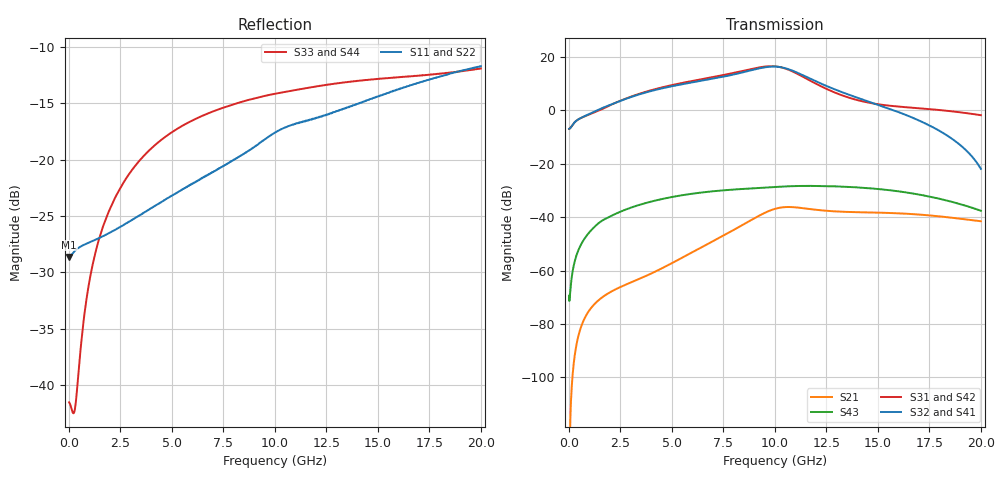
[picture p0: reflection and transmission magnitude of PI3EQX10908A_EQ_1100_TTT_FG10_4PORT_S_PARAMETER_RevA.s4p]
! NPort=4 DATA=2000 NOISE=0 GROUPDELAY=0 COMPLEX_DATAFORMAT=POLAR
! NumOfBlock=1 NumOfParam=0
! .MODEL Smodel S TSTONEFILE=PI3EQX10908A_EQ_1100_TTT_FG10_4PORT_S_PARAMETER_RevA.s4p TYPE=S
!  -- The above .MODEL line can be used for the S element in the netlist.
! The s parameter is extracted from the linear redriver, it is not bi-directional; only s(4,1)s(4,2) and s(3,1)s(3,2)
! should be the insertion loss
!Port definition:
!Port1 = input+
!Port2 = input-
!Port3 = output+
!Port4 = output-
# Hz S MA R  50
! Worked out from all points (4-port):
!   2000 points, 10 MHz to 20 GHz, reference 50 ohm
!   strongest paths, dB at 10 MHz, 5.01 GHz, 10.01 GHz, 15.01 GHz, 20 GHz:
!     S32: -6.9, 9.0, 16.4, 2.1, -21.9
!     S41: -6.9, 9.0, 16.4, 2.1, -21.9
!     S31: -6.9, 9.5, 16.5, 2.3, -1.8
!     S42: -6.9, 9.5, 16.5, 2.3, -1.8
!     S43: -69.4, -32.4, -28.7, -29.5, -37.6
!     S21: -127.3, -57.2, -36.9, -38.3, -41.5
!   lowest |S11| = -28.6 dB at 10 MHz (marker M1), VSWR 1.08, Z = 46.4 - j0.024 ohm
!   |S11| at or under -10 dB: start of sweep to end of sweep
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1e7  0.03701 -179.6  4.34e-07 14.6  0 0.0  0 0.0
     4.34e-07 14.6  0.03701 -179.6  0 0.0  0 0.0
     0.4506 1.2  0.4506 -178.8  0.008374 26.0  0.00034 -27.1
     0.4506 -178.8  0.4506 1.2  0.00034 -27.1  0.008374 26.0
6.56e9  0.08394 -120.5  0.002887 132.8  3.443e-07 66.5  1.859e-07 138.2
        0.002887 132.8  0.08396 -120.5  1.859e-07 138.2  3.444e-07 66.5
        3.905 -50.0  3.644 123.5  0.1577 13.6  0.0293 18.3
        3.644 123.6  3.905 -50.0  0.0293 18.3  0.1577 13.6
9.05e9  0.1146 -111.9  0.009735 109.4  2.357e-06 20.8  1.48e-06 114.5
        0.00974 109.5  0.1147 -111.9  1.481e-06 114.5  2.357e-06 20.8
        6.169 -111.9  5.875 62.4  0.1876 -6.2  0.03483 -7.5
        5.876 62.4  6.17 -111.9  0.03483 -7.5  0.1876 -6.2
1.03e10  0.1363 -112.2  0.01515 72.4  4.098e-06 -13.3  4.299e-06 81.0
         0.01515 72.5  0.1364 -112.2  4.302e-06 81.0  4.099e-06 -13.4
         6.388 -164.8  6.407 8.7  0.1984 -14.6  0.03723 -20.2
         6.407 8.7  6.389 -164.8  0.03723 -20.2  0.1984 -14.6
1.142e10  0.1477 -113.5  0.01464 41.2  5.012e-06 -24.1  7.504e-06 44.2
          0.01463 41.2  0.1477 -113.5  7.507e-06 44.2  5.01e-06 -24.1
          4.135 153.6  4.43 -36.2  0.207 -21.1  0.03845 -33.6
          4.43 -36.2  4.135 153.6  0.03845 -33.6  0.207 -21.1
1.361e10  0.1721 -111.9  0.0125 13.7  1.37e-05 -36.3  1.641e-05 -5.6
          0.01249 13.7  0.1722 -111.9  1.642e-05 -5.6  1.369e-05 -36.3
          1.718 123.3  1.95 -84.2  0.2216 -32.5  0.03678 -60.1
          1.95 -84.2  1.718 123.4  0.03678 -60.1  0.2216 -32.5
2e10  0.26 -114.9  0.008386 -40.1  8.854e-05 -147.9  7.175e-05 -139.1
      0.008381 -39.8  0.2602 -114.9  7.177e-05 -139.1  8.852e-05 -147.9
      0.8111 53.5  0.07998 169.6  0.2539 -52.2  0.01317 -136.6
      0.08054 170.2  0.8121 53.5  0.01317 -136.6  0.2539 -52.2
